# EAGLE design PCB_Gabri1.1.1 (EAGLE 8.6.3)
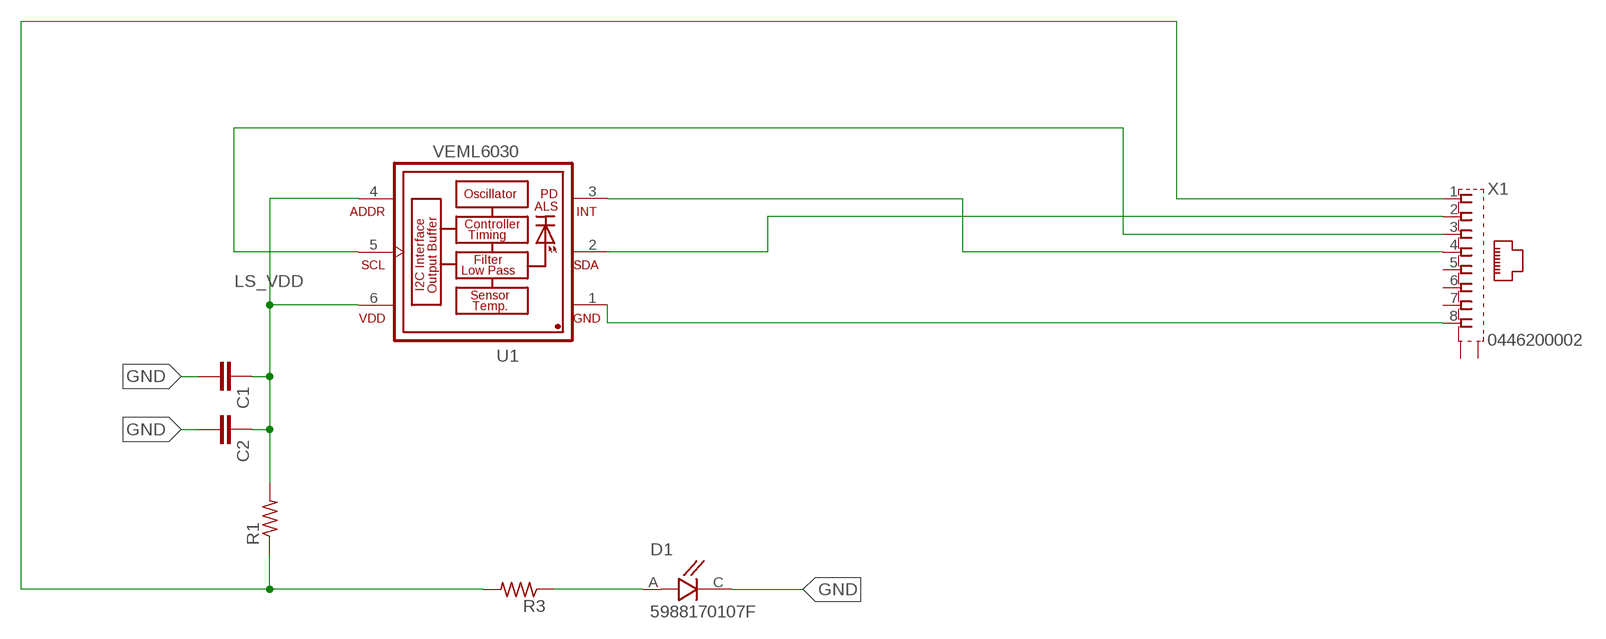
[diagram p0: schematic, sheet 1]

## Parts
C1  C-EU025-024X044  [C025-024X044]
C2  C-EU025-024X044  [C025-024X044]
D1  5988170107F  [LEDC2012X70N]
R1  R-US_R0805  [R0805]
R3  R-US_R0805  [R0805]
U1  VEML6030  [VISHAY_VEML6030_2X2X0.87]
X1  0446200002  [0446200002]

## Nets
3V3: R1.1 R3.2 X1.1
GND: C1.2 C2.2 D1.C U1.1(GND) X1.8
INT: U1.3(INT) X1.4
LS_VDD: C1.1 C2.1 R1.2 U1.4(ADDR) U1.6(VDD)
N$1: D1.A R3.1
SCL: U1.5(SCL) X1.3
SDA: U1.2(SDA) X1.2
Unconnected: X1.5 X1.6 X1.7 X1.S@1(S1) X1.S@2(S2)

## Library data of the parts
C1 C2 = resistor:C-EU: CAPACITOR, European symbol
D1 = 5988170107F:5988170107F: Standard LEDs - SMD Green Water Clr 40mcd 570nm; AVAILABILITY: Unavailable; DESCRIPTION: LED GREEN CLEAR 0805 SMD; MF: Dialight; MP: 5988170107F; PACKAGE: 0805 Dialight; PRICE: None
R1 R3 = resistor:R-US_: RESISTOR, American symbol
U1 = VEML6030:VEML6030: VEML6030 High Accuracy Ambient Light Sensor with I2C Interface: VEML6030 is a high accuracy ambient light digital 16-bit resolution sensor in a miniature transparent 2 mm x 2 mm package. It includes a high sensitive photodiode, a low noise amplifier, a 16-bit A/D converter and supports an easy to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; AVAILABILITY: Unavailable; DESCRIPTION: VEML6030 Series 2 x 2 x 0.85 mm 50 mW I2C High Accuracy Ambient Light Sensor; MF: Vishay; MP: VEML6030; PACKAGE: SMD-6 Vishay; PRICE: None
X1 = 0446200002:0446200002: RJ-45 INVERTED MODULAR JACK ASSEMBLY WITH RJ-11 KEEPOUT FEATURE Source: Data sheet MOLEX 0446200002 BUCHSE, RJ45, GESCHIRMT Source: Farnell; AVAILABILITY: Unavailable; DESCRIPTION: Conn RJ-45 RCP 8 POS 2.04mm Solder RA Thru-Hole 8 Terminal 1 Port Tray Cat 3; MF: Molex, LLC; MP: 0446200002; PACKAGE: None; PRICE: None

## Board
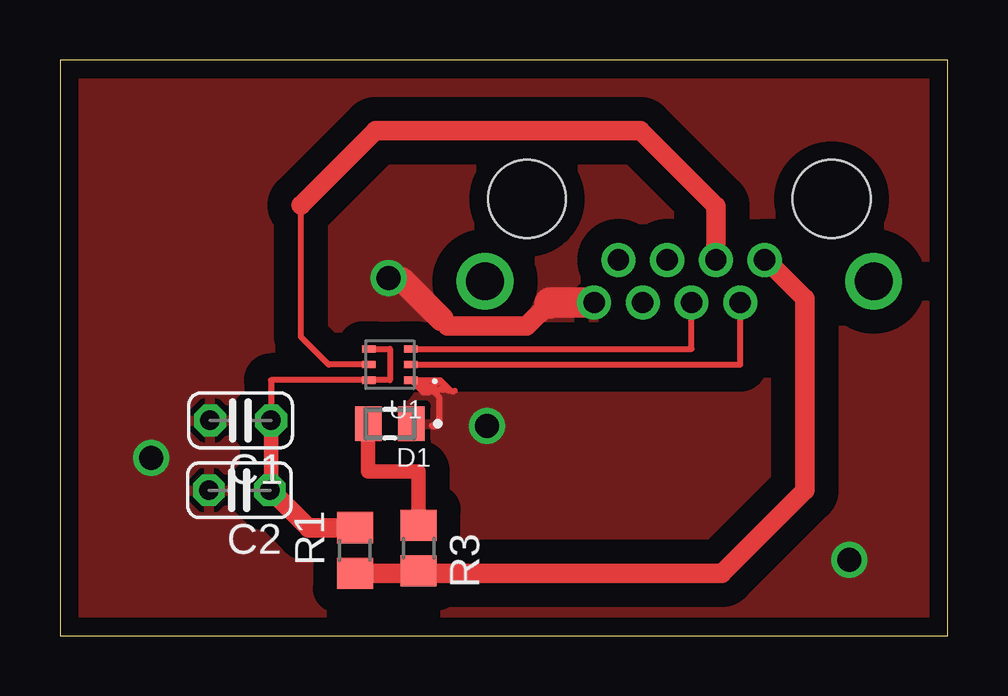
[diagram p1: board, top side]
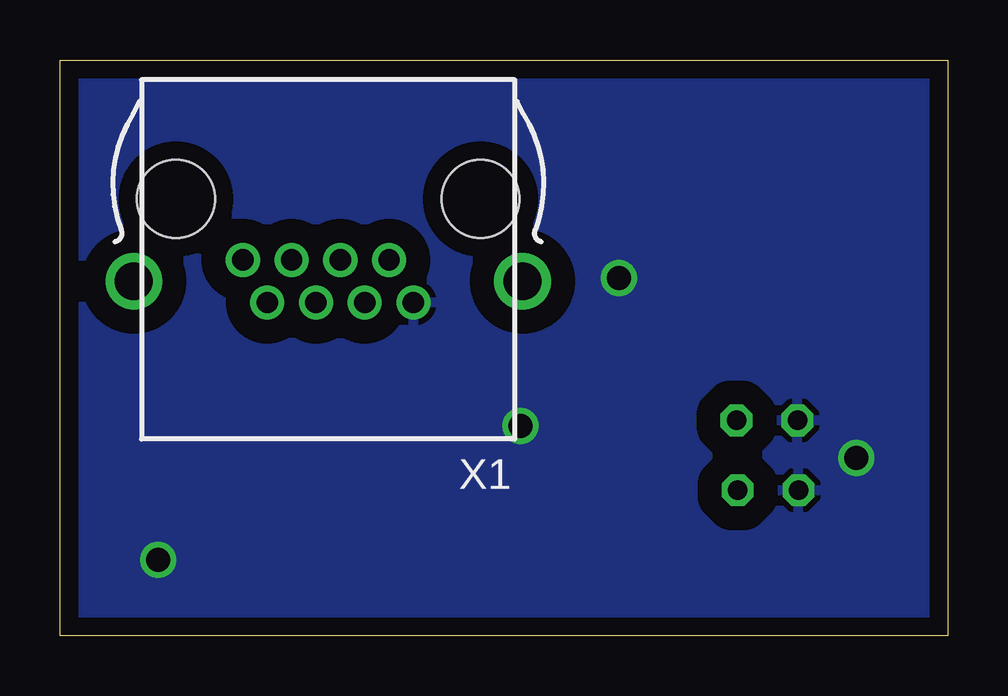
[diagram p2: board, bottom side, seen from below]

Size 37 x 24 mm. Coordinates in mm from the lower left corner, seen from the top.
Outline: 0,0 37,0 37,24 0,24 0,0
Copper layers (1*16): Top 0.035mm / dielectric 1.5mm / Bottom 0.035mm
Design rules "default *": minimum track width 10mil, minimum drill 0.5mm, track to track 1mm, track to pad 1mm, pad to pad 1mm, via to via 1mm, smd to smd 0.8mm, copper to edge 30mil, drill to drill 8mil, minimum pad ring 10mil, minimum via ring 8mil, stop-mask expansion 4mil, vias tented up to drill 0mil, thermal gap 10mil

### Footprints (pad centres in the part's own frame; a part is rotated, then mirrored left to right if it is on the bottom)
C025-024X044 = drill 0.813 octagon: 1 -1.27,0; 2 1.27,0
LEDC2012X70N = smd 1.1 x 1.45: A 0.9,0; C -0.9,0
R0805 = smd 1.3 x 1.5: 1 -0.95,0; 2 0.95,0
VISHAY_VEML6030_2X2X0.87 = smd 0.55 x 0.3: 1 -0.875,0.65; 2 -0.875,0; 3 -0.875,-0.65; 4 0.875,-0.65; 5 0.875,0; 6 0.875,0.65
0446200002 = drill 0.889 pad 1.422: 1 3.556,2.54; 2 2.54,4.318; 3 1.524,2.54; 4 0.508,4.318; 5 -0.508,2.54; 6 -1.524,4.318; 7 -2.54,2.54; 8 -3.556,4.318 | drill 1.575 pad 2.286: S@1 -8.103,3.429; S@2 8.103,3.429 | hole 3.251: 6.35,0; -6.35,0

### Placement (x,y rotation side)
C1  7.53,8.97 180 top
C2  7.48,6.06 180 top
D1  13.75,8.83 180 top
R1  12.3,3.55 90 top
R3  14.95,3.65 270 top
U1  13.75,11.3 180 top
X1  25.82,18.2 180 bottom

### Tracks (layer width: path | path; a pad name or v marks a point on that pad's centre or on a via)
3V3
  Top 0.254: X1.1 29.41,15.69
  Top 0.813: R1.1 14.95,2.6 | 14.95,2.6 R3.2 | 29.41,15.69 31.05,14.05 31.05,6.05 27.6,2.6 14.95,2.6
GND  (via drill 1)
  Top 0.254: U1.1 15.12,10.15 15.4,10.15 | 15.6,10.15 15.4,10.15 | U1.1 14.9,10.65 15.4,10.15 | U1.1 15.1,10.65 | 15.1,10.65 15.55,10.2 | 15.55,10.2 15.6,10.15 | 15.1,10.65 15.5,10.65 | 15.5,10.65 15.85,10.65 16.03,10.47 | 15.5,10.65 15.55,10.6 15.55,10.2 | 15.8,10.6 15.6,10.4 15.6,10.15 | 16.03,10.47 16.3,10.2 | 16.3,10.2 16.45,10.2 | 16.3,10.2 16.2,10.2 16.15,10.25 15.8,10.25 | 16.03,10.47 15.7,10.15 15.6,10.15 | 15.6,10.15 15.8,9.95 15.8,8.75 15.65,8.75 15.6,8.7 15.55,8.7 15.5,8.75 | 14.5,14.9 v13.7,14.9
  Top 0.813: 16,13.05 16.15,12.9 19.45,12.9 20.4,13.85
  Top 1.016: 13.65,14.85 14.25,14.85 15.9,13.2
  Top 1.27: X1.8 20.43,13.88 20.4,13.85
  other vias: 17.8,8.75 32.9,3.15 3.8,7.4
  pour Bottom: 0.25,23.8 0.25,0.25 36.85,0.25 36.85,23.8
  pour Top: 0.4,23.55 0.4,0.35 36.6,0.35 36.6,23.55
INT
  Top 0.254: U1.3 26.33,11.95 X1.4
LS_VDD
  Top 0.254: C1.1 8.8,10.65 U1.6 13.75,10.65 13.75,11.95 U1.4
  Top 0.61: C1.1 8.8,6.06 C2.1
  Top 0.813: R1.2 10.36,4.5 8.8,6.06
N$1
  Top 0.61: D1.A 12.85,6.85 14.95,6.85 R3.1
SCL
  Top 0.254: U1.5 11.2,11.3 10.05,12.45 10.05,17.95
  Top 0.813: X1.3 27.34,17.91 24.2,21.05 13.15,21.05 10.05,17.95
SDA
  Top 0.254: U1.2 28.36,11.3 X1.2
